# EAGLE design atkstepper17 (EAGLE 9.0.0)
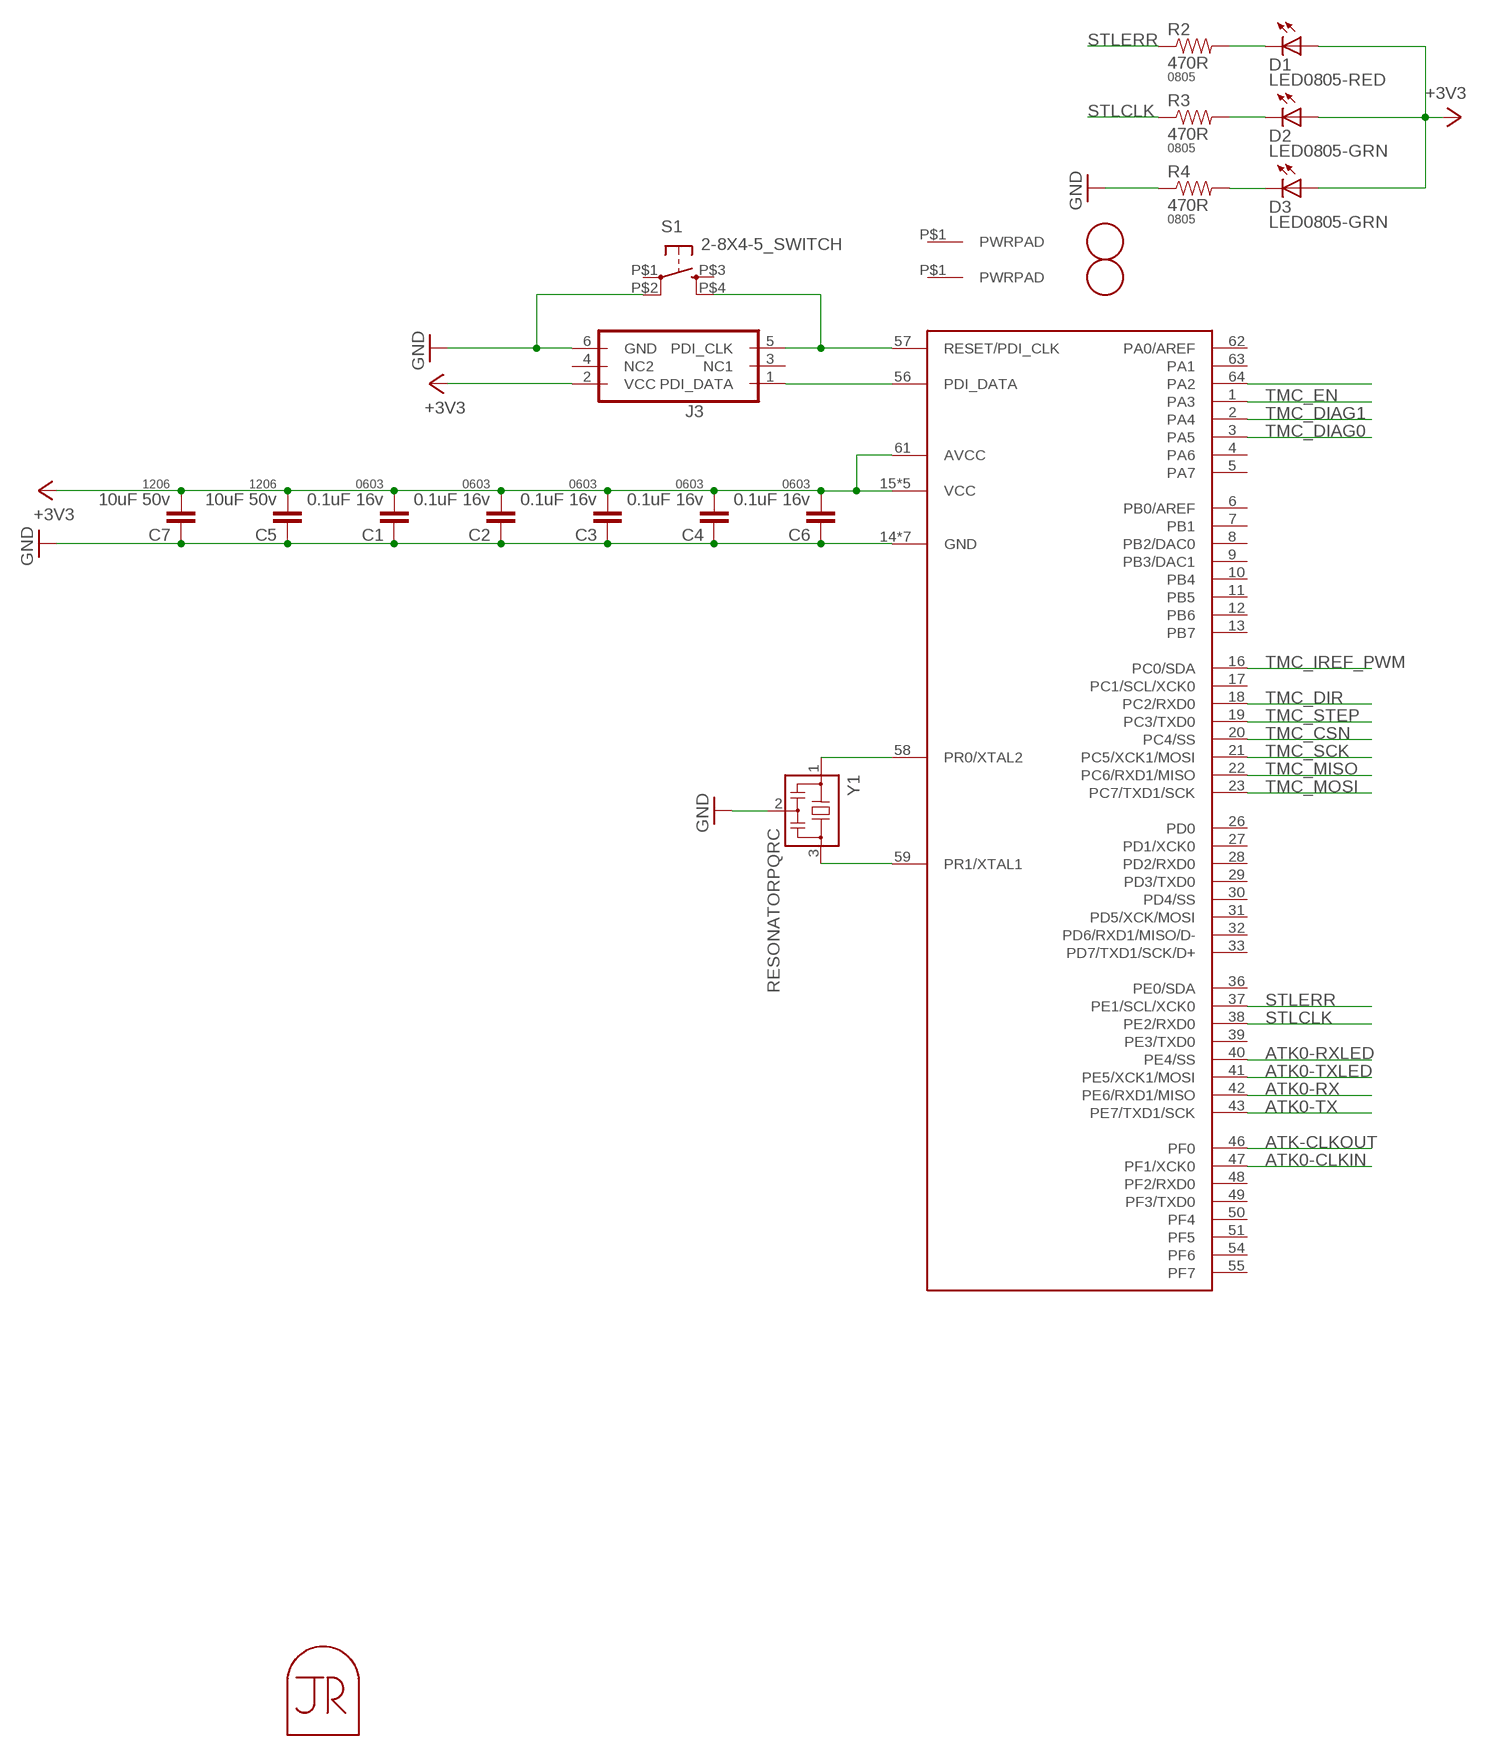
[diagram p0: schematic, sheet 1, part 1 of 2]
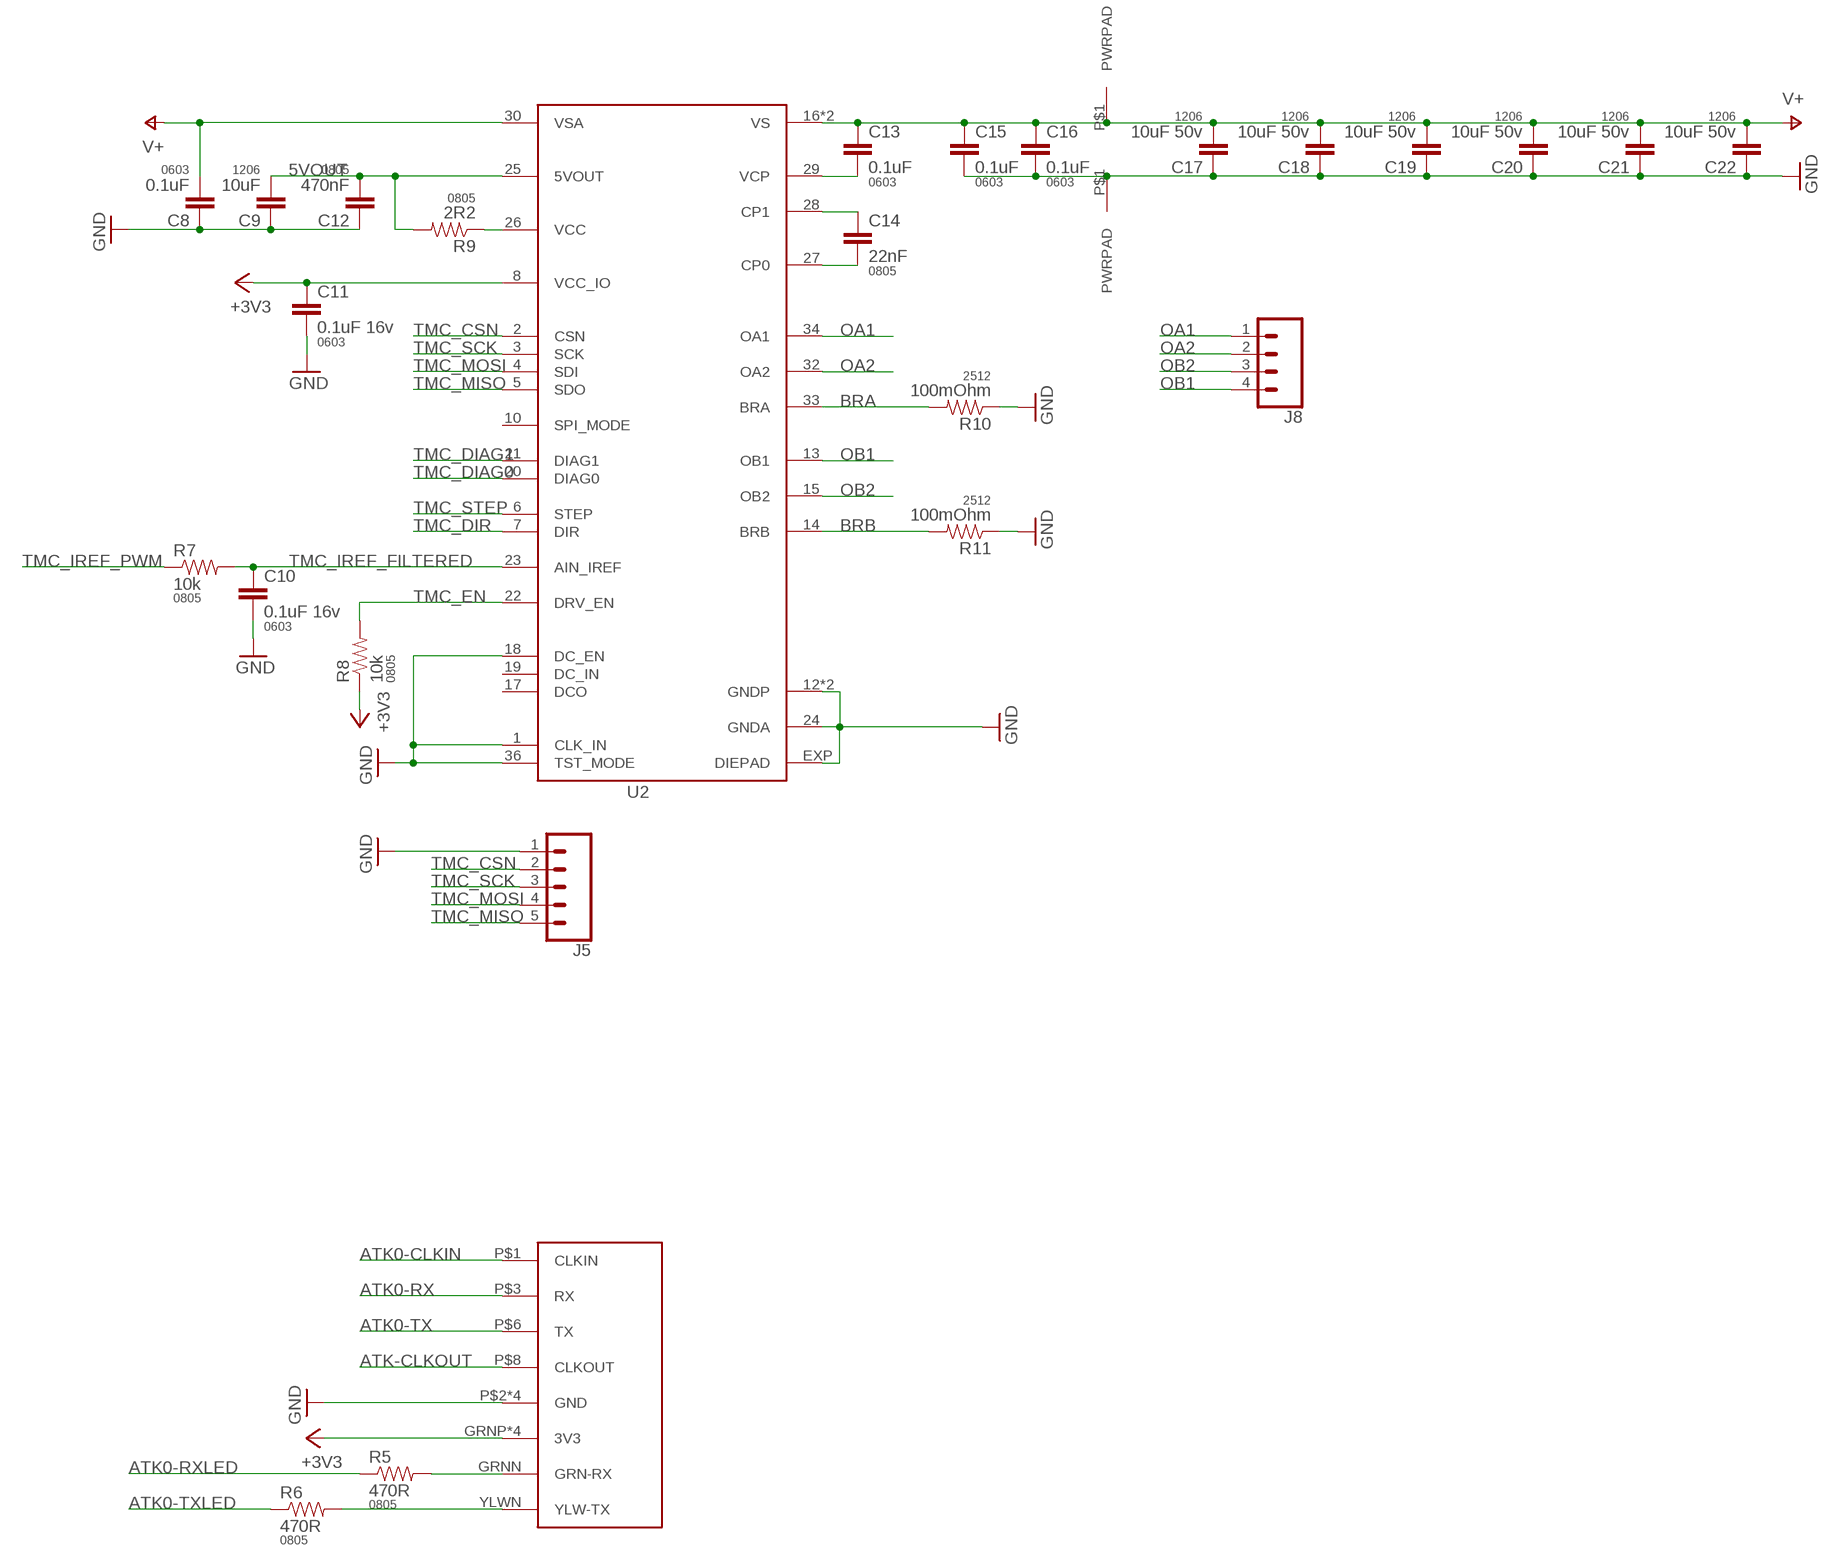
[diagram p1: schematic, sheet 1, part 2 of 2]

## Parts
C1  0.1uF 16v  CAP0603-CAP  [0603-CAP]
C2  0.1uF 16v  CAP0603-CAP  [0603-CAP]
C3  0.1uF 16v  CAP0603-CAP  [0603-CAP]
C4  0.1uF 16v  CAP0603-CAP  [0603-CAP]
C5  10uF 50v  CAP1206  [1206]
C6  0.1uF 16v  CAP0603-CAP  [0603-CAP]
C7  10uF 50v  CAP1206  [1206]
C8  0.1uF  CAP0603-CAP  [0603-CAP]
C9  10uF  CAP1206  [1206]
C10  0.1uF 16v  CAP0603-CAP  [0603-CAP]
C11  0.1uF 16v  CAP0603-CAP  [0603-CAP]
C12  470nF  CAP0805  [0805]
C13  0.1uF  CAP0603-CAP  [0603-CAP]
C14  22nF  CAP0805  [0805]
C15  0.1uF  CAP0603-CAP  [0603-CAP]
C16  0.1uF  CAP0603-CAP  [0603-CAP]
C17  10uF 50v  CAP1206  [1206]
C18  10uF 50v  CAP1206  [1206]
C19  10uF 50v  CAP1206  [1206]
C20  10uF 50v  CAP1206  [1206]
C21  10uF 50v  CAP1206  [1206]
C22  10uF 50v  CAP1206  [1206]
D1  LED0805-RED  LED0805  [LED0805]
D2  LED0805-GRN  LED0805  [LED0805]
D3  LED0805-GRN  LED0805  [LED0805]
J1  PWRPADM3  [PWRPAD_3-25MM]
J2  PWRPADM3  [PWRPAD_3-25MM]
J3  PDIFEMALE_SMD  [PDI_2X3_SMD]
J4  ATK-PHY  [RJ45-LED-RJE7318800XXX]
J5  CONN_05NO_SILK  [1X05_NO_SILK]
J6  PWRPAD  [PWRPAD_M3-PEM-MOUNT]
J7  PWRPAD  [PWRPAD_M3-PEM-MOUNT]
J8  CONN_04LONGPADS  [1X04_LONGPADS]
MP1  JRTOMBSTONE  [JRTOMBSTONE]
R2  470R  RESISTOR0805-RES  [0805]
R3  470R  RESISTOR0805-RES  [0805]
R4  470R  RESISTOR0805-RES  [0805]
R5  470R  RESISTOR0805-RES  [0805]
R6  470R  RESISTOR0805-RES  [0805]
R7  10k  RESISTOR0805-RES  [0805]
R8  10k  RESISTOR0805-RES  [0805]
R9  2R2  RESISTOR0805-RES  [0805]
R10  100mOhm  RESISTOR2512  [R2512]
R11  100mOhm  RESISTOR2512  [R2512]
S1  2-8X4-5_SWITCH  [TACT-SWITCH-KMR6]
U1  ATXMEGA_A3UQFN  [QFN-64-9X9MM]
U2  TMC2130  [QFN36-5X6]
U$1  FIDUCIAL  [FIDUCIAL_1MM]
U$2  FIDUCIAL  [FIDUCIAL_1MM]
Y1  RESONATORPQRC  [RES_PRQC]

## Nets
5VOUT: C9.2 C12.2 R9.2 U2.25(5VOUT)
+3V3: C1.2 C2.2 C3.2 C4.2 C5.2 C6.2 C7.2 C11.1 D1.1(A) D2.1(A) D3.1(A) J3.2(VCC) J4.GRNP(3V3) J4.P$4(3V3) J4.P$5(3V3) J4.YLWP(3V3) R8.1 U1.15(VCC) U1.25(VCC) U1.35(VCC) U1.45(VCC) U1.53(VCC) U1.61(AVCC) U2.8(VCC_IO)
ATK0-CLKIN: J4.P$1(CLKIN) U1.47(PF1/XCK0)
ATK0-RX: J4.P$3(RX) U1.42(PE6/RXD1/MISO)
ATK0-RXLED: R5.1 U1.40(PE4/SS)
ATK0-TX: J4.P$6(TX) U1.43(PE7/TXD1/SCK)
ATK0-TXLED: R6.1 U1.41(PE5/XCK1/MOSI)
ATK-CLKOUT: J4.P$8(CLKOUT) U1.46(PF0)
BRA: R10.2 U2.33(BRA)
BRB: R11.2 U2.14(BRB)
GND: C1.1 C2.1 C3.1 C4.1 C5.1 C6.1 C7.1 C8.1 C9.1 C10.2 C11.2 C12.1 C15.2 C16.2 C17.1 C18.1 C19.1 C20.1 C21.1 C22.1 J3.6(GND) J4.P$2(GND) J4.P$7(GND) J4.SHDL1(GND) J4.SHDL2(GND) J5.1 J7.P$1(PWRPAD) R4.1 R10.1 R11.1 S1.P$2(P1) U1.14(GND) U1.24(GND) U1.34(GND) U1.44(GND) U1.52(GND) U1.60(GND) U1.P$1(GND) U2.1(CLK_IN) U2.12(GNDP) U2.18(DC_EN) U2.24(GNDA) U2.35(GNDP) U2.36(TST_MODE) U2.EXP(DIEPAD) Y1.2
N$1: D3.2(C) R4.2
N$2: J3.5(PDI_CLK) S1.P$4(S1) U1.57(RESET/PDI_CLK)
N$3: U1.58(PR0/XTAL2) Y1.1
N$4: U1.59(PR1/XTAL1) Y1.3
N$5: D2.2(C) R3.2
N$6: D1.2(C) R2.2
N$8: J3.1(PDI_DATA) U1.56(PDI_DATA)
N$12: C14.2 U2.27(CP0)
N$13: R9.1 U2.26(VCC)
N$14: C14.1 U2.28(CP1)
N$15: C13.2 U2.29(VCP)
N$16: J4.GRNN(GRN-RX) R5.2
N$17: J4.YLWN(YLW-TX) R6.2
N$18: U1.64(PA2)
OA1: J8.1 U2.34(OA1)
OA2: J8.2 U2.32(OA2)
OB1: J8.4 U2.13(OB1)
OB2: J8.3 U2.15(OB2)
STLCLK: R3.1 U1.38(PE2/RXD0)
STLERR: R2.1 U1.37(PE1/SCL/XCK0)
TMC_CSN: J5.2 U1.20(PC4/SS) U2.2(CSN)
TMC_DIAG0: U1.3(PA5) U2.20(DIAG0)
TMC_DIAG1: U1.2(PA4) U2.21(DIAG1)
TMC_DIR: U1.18(PC2/RXD0) U2.7(DIR)
TMC_EN: R8.2 U1.1(PA3) U2.22(DRV_EN)
TMC_IREF_FILTERED: C10.1 R7.2 U2.23(AIN_IREF)
TMC_IREF_PWM: R7.1 U1.16(PC0/SDA)
TMC_MISO: J5.5 U1.22(PC6/RXD1/MISO) U2.5(SDO)
TMC_MOSI: J5.4 U1.23(PC7/TXD1/SCK) U2.4(SDI)
TMC_SCK: J5.3 U1.21(PC5/XCK1/MOSI) U2.3(SCK)
TMC_STEP: U1.19(PC3/TXD0) U2.6(STEP)
V+: C8.2 C13.1 C15.1 C16.1 C17.2 C18.2 C19.2 C20.2 C21.2 C22.2 J6.P$1(PWRPAD) U2.16(VS) U2.30(VSA) U2.31(VS)
Unconnected: J1.P$1(PWRPAD) J2.P$1(PWRPAD) J3.3(NC1) J3.4(NC2) S1.P$1(P) S1.P$3(S) U1.4(PA6) U1.5(PA7) U1.6(PB0/AREF) U1.7(PB1) U1.8(PB2/DAC0) U1.9(PB3/DAC1) U1.10(PB4) U1.11(PB5) U1.12(PB6) U1.13(PB7) U1.17(PC1/SCL/XCK0) U1.26(PD0) U1.27(PD1/XCK0) U1.28(PD2/RXD0) U1.29(PD3/TXD0) U1.30(PD4/SS) U1.31(PD5/XCK/MOSI) U1.32(PD6/RXD1/MISO/D-) U1.33(PD7/TXD1/SCK/D+) U1.36(PE0/SDA) U1.39(PE3/TXD0) U1.48(PF2/RXD0) U1.49(PF3/TXD0) U1.50(PF4) U1.51(PF5) U1.54(PF6) U1.55(PF7) U1.62(PA0/AREF) U1.63(PA1) U2.10(SPI_MODE) U2.17(DCO) U2.19(DC_IN)

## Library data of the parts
C1-C4 C6 C8 C10 C11 C13 C15 C16 = borkedlabs-passives:CAP: Capacitor; PACKAGE: 0603
C5 C7 C9 C17-C22 = borkedlabs-passives:CAP: Capacitor; PACKAGE: 1206
C12 C14 = borkedlabs-passives:CAP: Capacitor; PACKAGE: 0805
D1-D3 = lights:LED: LED
J1 J2 J6 J7 = power:PWRPAD
J3 = microcontrollers:PDI: Multi connection point. Often used as Generic Header-pin footprint for 0.1 inch spaced/style header connections You can populate with any combo of single row headers, but if you'd like an exact match, check these: Header - 2x3 (Male, 0.1") (PRT-12807) Header - 2x3 (Female, 0.1") (PRT-13010) 2x3 Pin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; PROD_ID: CONN-11290
J4 = connector:ATK-PHY
J5 = SparkFun-Connectors:CONN_05: Multi connection point. Often used as Generic Header-pin footprint for 0.1 inch spaced/style header connections On any of the 0.1 inch spaced packages, you can populate with these: Break Away Headers - Straight (PRT-00116) Break Away Male Headers - Right Angle (PRT-00553) Female Headers (PRT-00115)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
J8 = SparkFun-Connectors:CONN_04: Multi connection point. Often used as Generic Header-pin footprint for 0.1 inch spaced/style header connections On any of the 0.1 inch spaced packages, you can populate with these: Break Away Headers - Straight (PRT-00116) Break Away Male Headers - Right Angle (PRT-00553) Female Headers (PRT-00115)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; PROD_ID: CONN-09696
MP1 = connector:JRTOMBSTONE
R2-R9 = borkedlabs-passives:RESISTOR: Resistor; PACKAGE: 0805
R10 R11 = borkedlabs-passives:RESISTOR: Resistor; PACKAGE: 2512
S1 = fab:2-8X4-5_SWITCH
U1 = microcontrollers:ATXMEGA_A3U
U2 = power:TMC2130
U$1 U$2 = connector:FIDUCIAL: For use by pick and place machines to calibrate the vision/machine, 1mm
Y1 = passives:RESONATOR

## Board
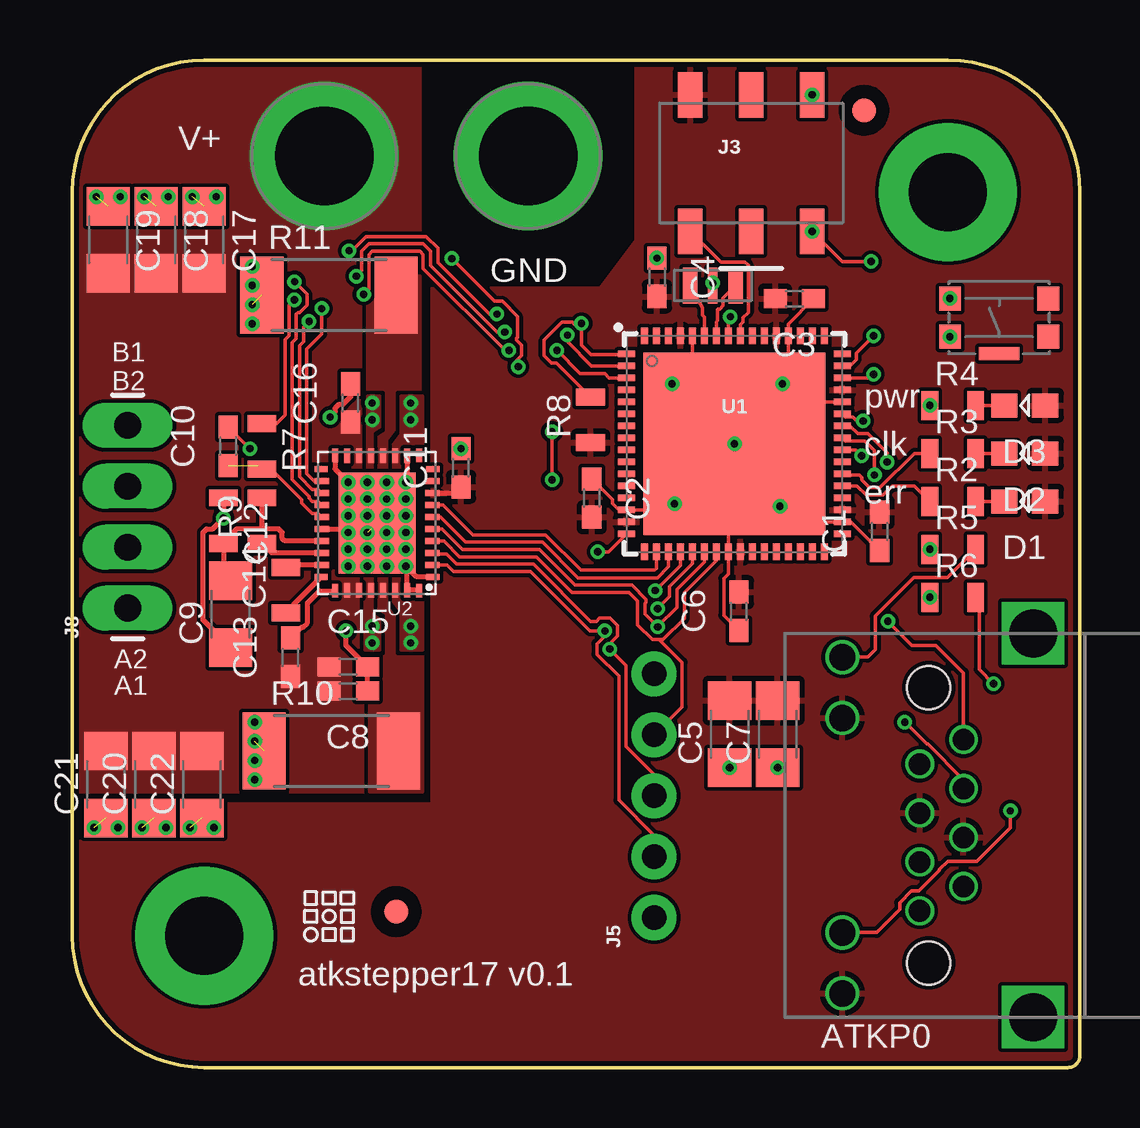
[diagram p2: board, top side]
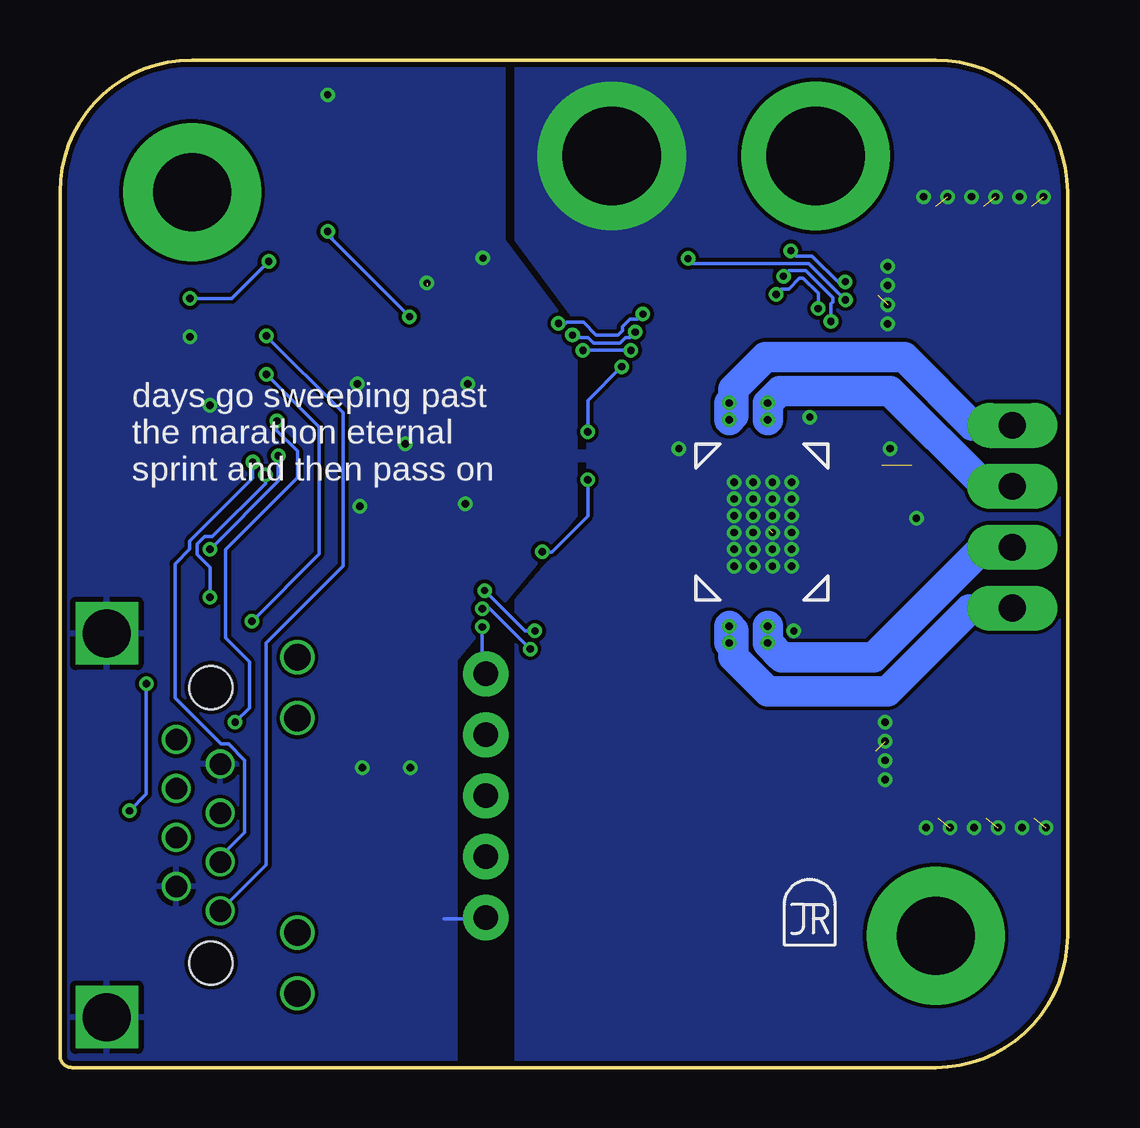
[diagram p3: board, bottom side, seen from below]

Size 42 x 42 mm. Coordinates in mm from the lower left corner, seen from the top.
Outline: 36.5,42 5.5,42 arc90 0,36.5 0,5.5 arc90 5.5,0 41.5,0 arc90 42,0.5 42,36.5 arc90 36.5,42
Copper layers (1*16): Top 0.035mm / dielectric 1.5mm / Bottom 0.035mm
Design rules "default *": minimum track width 6mil, minimum drill 0.3mm, track to track 6mil, track to pad 6mil, pad to pad 6mil, via to via 6mil, smd to smd 6mil, copper to edge 8mil, drill to drill 8mil, minimum pad ring 6mil, minimum via ring 6mil, stop-mask expansion 4mil, vias tented up to drill 27mil, thermal gap 9mil

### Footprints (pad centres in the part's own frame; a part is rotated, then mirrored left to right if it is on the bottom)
0603-CAP = smd 0.96 x 0.8: 1 -0.8,0; 2 0.8,0
1206 = smd 1.6 x 1.8: 1 -1.4,0; 2 1.4,0
0805 = smd 0.7 x 1.2: 1 -0.95,0; 2 0.95,0
LED0805 = smd 1.1 x 1: 1 -0.85,0; 2 0.85,0
PWRPAD_3-25MM = drill 3.25 pad 5.75: P$1 0,0
PDI_2X3_SMD = smd 1.02 x 1.9: 1 -2.54,-2.85; 2 -2.54,2.85; 3 0,-2.85; 4 0,2.85; 5 2.54,-2.85; 6 2.54,2.85
RJ45-LED-RJE7318800XXX = drill 1.1: GRNN 7.01,3.6; GRNP 4.47,3.6; YLWN -4.47,3.6; YLWP -7.01,3.6 | drill 0.9: P$1 -3.57,0.38; P$2 -2.55,-1.45; P$3 -1.53,0.38; P$4 -0.51,-1.45; P$5 0.51,0.38; P$6 1.53,-1.45; P$7 2.55,0.38; P$8 3.57,-1.45 | drill 2 square: SHDL1 -8,-4.35; SHDL2 8,-4.35 | hole 1.8: -5.74,0; 5.74,0
1X05_NO_SILK = drill 1.016 pad 1.88: 1 0,0; 2 2.54,0; 3 5.08,0; 4 7.62,0; 5 10.16,0
PWRPAD_M3-PEM-MOUNT = drill 4.1 pad 6.2: P$1 0,0
1X04_LONGPADS = drill 1.118 pad 1.88 long: 1 0,0; 2 2.54,0; 3 5.08,0; 4 7.62,0
R2512 = smd 1.8 x 3.2: 1 -2.8,0; 2 2.8,0
TACT-SWITCH-KMR6 = smd 0.9 x 1: P$1 -2.05,0.8; P$2 2.05,0.8; P$3 -2.05,-0.8; P$4 2.05,-0.8 | smd 1.7 x 0.55: P$5 0,1.5
QFN-64-9X9MM = smd 0.7 x 0.275: 1 -4.5,3.75; 2 -4.5,3.25; 3 -4.5,2.75; 4 -4.5,2.25; 5 -4.5,1.75; 6 -4.5,1.25; 7 -4.5,0.75; 8 -4.5,0.25; 9 -4.5,-0.25; 10 -4.5,-0.75; 11 -4.5,-1.25; 12 -4.5,-1.75; 13 -4.5,-2.25; 14 -4.5,-2.75; 15 -4.5,-3.25; 16 -4.5,-3.75; 33 4.5,-3.75; 34 4.5,-3.25; 35 4.5,-2.75; 36 4.5,-2.25; 37 4.5,-1.75; 38 4.5,-1.25; 39 4.5,-0.75; 40 4.5,-0.25; 41 4.5,0.25; 42 4.5,0.75; 43 4.5,1.25; 44 4.5,1.75; 45 4.5,2.25; 46 4.5,2.75; 47 4.5,3.25; 48 4.5,3.75 | smd 0.275 x 0.7: 17 -3.75,-4.5; 18 -3.25,-4.5; 19 -2.75,-4.5; 20 -2.25,-4.5; 21 -1.75,-4.5; 22 -1.25,-4.5; 23 -0.75,-4.5; 24 -0.25,-4.5; 25 0.25,-4.5; 26 0.75,-4.5; 27 1.25,-4.5; 28 1.75,-4.5; 29 2.25,-4.5; 30 2.75,-4.5; 31 3.25,-4.5; 32 3.75,-4.5; 49 3.75,4.5; 50 3.25,4.5; 51 2.75,4.5; 52 2.25,4.5; 53 1.75,4.5; 54 1.25,4.5; 55 0.75,4.5; 56 0.25,4.5; 57 -0.25,4.5; 58 -0.75,4.5; 59 -1.25,4.5; 60 -1.75,4.5; 61 -2.25,4.5; 62 -2.75,4.5; 63 -3.25,4.5; 64 -3.75,4.5 | smd 7.6 x 7.6: P$1 0,0
QFN36-5X6 = smd 0.55 x 0.25: 1 -2.325,1.75; 10 -2.325,-2.75; 19 2.325,-2.75; 28 2.325,1.75 | smd 0.6 x 0.25: 2 -2.3,1.25; 3 -2.3,0.75; 4 -2.3,0.25; 5 -2.3,-0.25; 6 -2.3,-0.75; 7 -2.3,-1.25; 8 -2.3,-1.75; 9 -2.3,-2.25; 20 2.3,-2.25; 21 2.3,-1.75; 22 2.3,-1.25; 23 2.3,-0.75; 24 2.3,-0.25; 25 2.3,0.25; 26 2.3,0.75; 27 2.3,1.25 | smd 0.25 x 0.55: 11 -1.75,-3.325; 18 1.75,-3.325; 29 1.75,2.325; 36 -1.75,2.325 | smd 0.25 x 0.6: 12 -1.25,-3.3; 13 -0.75,-3.3; 14 -0.25,-3.3; 15 0.25,-3.3; 16 0.75,-3.3; 17 1.25,-3.3; 30 1.25,2.3; 31 0.75,2.3; 32 0.25,2.3; 33 -0.25,2.3; 34 -0.75,2.3; 35 -1.25,2.3 | smd 3.2 x 4.2: EXP 0,-0.5
FIDUCIAL_1MM = smd 1 x 1: 1 0,0
RES_PRQC = smd 0.6 x 1.5: 1 -0.95,0; 3 0.95,0 | smd 0.4 x 1.5: 2 0,0

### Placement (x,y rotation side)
C1  33.65,22.35 90 top
C2  21.65,23.74 270 top
C3  30.1,32.05 180 top
C4  24.37,32.95 270 top
C5  27.4,13.9 90 top
C6  27.79,19.02 90 top
C7  29.4,13.9 90 top
C8  11.5,15.7 180 top
C9  6.6,18.9 90 top
C10  6.5,25.9 90 top
C11  16.2,25 90 top
C12  6.3,22.8 270 top
C13  9.1,17.1 90 top
C14  8.9,19.9 90 top
C15  11.5,16.7 0 top
C16  11.6,27.7 90 top
C17  5.5,34.5 270 top
C18  3.5,34.5 270 top
C19  1.5,34.5 270 top
C20  3.4,11.8 90 top
C21  1.4,11.8 90 top
C22  5.4,11.8 90 top
D1  39.7,23.6 180 top
D2  39.7,25.6 180 top
D3  39.7,27.6 180 top
J1  5.5,5.5 180 top
J2  36.5,36.5 180 top
J3  28.3,37.7 0 top
J4  35.7,10.1 90 top
J5  24.25,6.25 90 top
J6  10.5,38 180 top
J7  19,38 180 top
J8  2.3,19.15 90 top
MP1  10.7,6.1 0 bottom
R2  36.7,23.6 0 top
R3  36.7,25.6 0 top
R4  36.7,27.6 0 top
R5  36.7,21.6 0 top
R6  36.7,19.6 0 top
R7  7.9,25.9 270 top
R8  21.6,27 90 top
R9  7.9,22.8 90 top
R10  10.8,13.2 0 top
R11  10.7,32.2 0 top
S1  38.63,31.26 180 top
U1  27.6,26 0 top
U2  12.7,22.2 180 top
U$1  13.5,6.5 0 top
U$2  33,39.9 0 top
U$5  [CBA-SILK-LOGO]  10.7,6.3 90 top
Y1  26.7,32.6 180 top

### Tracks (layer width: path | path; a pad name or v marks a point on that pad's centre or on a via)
5VOUT
  Top 0.203: C12.2 6.2,21.65 | C12.2 6.3,21.9 6.85,22.45 7.9,22.45 | C12.2 6.3,20.6 C9.2 | U2.25 8.85,21.95 8.75,22.05 8.75,22.3 8.61,22.45 7.9,22.45 | R9.2 7.9,22.45
+3V3
  Top 0.203: U2.8 15.95,23.95 C11.1
  pour Top: -3,11 15,11 15,32.5 22,32.5 23.5,34.5 23.5,43 43,43 43,-2 -3,-2
ATK0-CLKIN  (via drill 0.3)
  Top 0.152: v33.4,30.5 32.68,29.78 32.68,29.52 32.41,29.25 U1.47
  Bottom 0.152: v33.4,30.5 30.2,27.3 30.2,20.9 33.4,17.7 33.4,8.45 J4.P$1
ATK0-RX  (via drill 0.3)
  Top 0.152: U1.42 32.41,26.75 32.74,26.42 33.17,26.42 33.97,25.62 v33.97,25.24
  Bottom 0.152: v33.97,25.24 33.97,24.57 36.59,21.95 36.59,21.61 37.2,21 37.2,15.4 35.28,13.48 34.98,13.48 34.3,12.8 34.3,9.8 35.32,8.78 J4.P$3
ATK0-RXLED  (via drill 0.3)
  Top 0.152: U1.40 32.66,25.75 v32.91,25.5
  Bottom 0.152: v32.91,25.5 32.91,24.45 R5.1
  other vias: 35.75,21.6
ATK0-TX  (via drill 0.3)
  Top 0.152: U1.43 32.23,27.12 32.55,27.12 32.71,26.95 v32.96,26.95 | v34.7,14.4 35.62,13.48 35.66,13.48 37.15,11.99 J4.P$6
  Bottom 0.152: v32.96,26.95 32.96,26.56 32.1,25.7 32.1,24.6 35.1,21.6 35.1,17.9 34.1,16.9 34.1,15 v34.7,14.4
ATK0-TXLED  (via drill 0.3)
  Top 0.152: U1.41 32.23,26.12 33.04,26.12 33.44,25.72 v33.44,24.7
  Bottom 0.152: v33.44,24.7 33.44,24.34 35.65,22.13 35.97,22.13 36.28,21.82 36.28,21.38 35.75,20.85 R6.1
  other vias: 35.75,19.6
ATK-CLKOUT  (via drill 0.3)
  Top 0.152: U1.46 33.25,28.75 v33.4,28.9 | v34,18.6 35,17.6 36,17.6 37.15,16.45 J4.P$8
  Bottom 0.152: v33.4,28.9 31.2,26.7 31.2,21.4 v34,18.6
BRA
  pour Top (rank 4, no thermals): 14.6,20.6 14.6,11.5 12.4,11.5 12.4,20.6
BRB
  pour Top (rank 4, no thermals): 14.5,33 14.5,23.9 12.3,23.9 12.3,33
GND  (via drill 0.3)  (10 unrouted)
  Top 0.152: 13.95,20.95 v13.9,20.9 | 13.95,23.95 U2.EXP | R4.1 35.85,27.7 | C10.2 v7.4,25.8 | U1.60 25.85,29.35 25.8,29.3 25.8,27.8 27.55,26.05 | 27.55,26.05 U1.P$1 27.45,25.85 | 29.45,27.95 29.85,28.35 U1.52 29.85,31 C3.1 | 29.45,27.95 27.55,26.05 | 27.35,25.75 v25.1,23.5 24.85,23.25 U1.14 22.79,23.25 22.52,23.52 22.52,23.67 C2.1 | 27.35,25.75 U1.24 27.35,20.58 27.16,20.39 27.16,18.85 C6.1 | 27.35,25.75 27.45,25.85 | 27.45,25.85 30.55,22.75 U1.34 32.45,22.75 C1.1 | U1.44 29.65,27.75 29.45,27.95
  Top 0.203: U2.24 12.45,22.45 U2.EXP | C9.1 5.45,18.65 5.45,22.3 5.59,22.45 5.85,22.45 v6.3,22.9 C12.1 | U2.12 13.95,24.45 v13.9,24.4 | 13.95,20.85 U2.35 14.43,19.9 U2.36 | 13.95,20.85 v13.9,20.9 | U2.1 14.35,20.45 13.95,20.85 | U2.18 10.95,24.95 v11.5,24.4 | C16.2 11.6,27.96 11.27,27.63 11.1,27.63 10.95,27.48 10.95,27.31 v10.74,27.11 | C8.1 C15.2 11.41,17.59 v11.41,18.2
  Bottom 0.152: J5.1 24.3,6.2 26,6.2
  other vias: 11.5,21.6 12.3,21.6 13.1,21.6 13.9,21.6 13.1,23.7 13.1,23 13.9,23.7 13.9,23 12.3,23 12.3,23.7 11.5,23.7 11.5,23 13.9,22.3 13.1,22.3 12.3,22.3 11.5,22.3 13.1,24.4 12.3,24.4 11.5,20.9 12.3,20.9 13.1,20.9 7.6,12 7.6,12.8 7.6,14.4 7.6,13.6 5.9,10 4.9,10 3.9,10 2.9,10 1.9,10 0.9,10 6,36.3 5,36.3 4,36.3 3,36.3 2,36.3 1,36.3 7.5,33.4 7.5,31 7.5,32.6 7.5,31.8 35.75,27.6 36.58,30.46 24.37,33.75 26.7,32.7 27.6,26 29.5,23.4 25,28.5 29.6,28.5 30.84,40.55 29.4,12.5 27.4,12.5 16.2,25.8
  pour Bottom: -2.5,-1.5 23,-1.5 23,19.5 20,23 20,25.3 20.5,25.3 20.5,25.7 20,25.7 20.1,30.6 23,34.5 23,44.5 -2.5,44.5
  pour Bottom: 25.5,-2.5 25.5,17 20.5,23 20.5,30.5 23.5,34.5 23.5,43 43.5,43 43.5,-2.5
N$1
  Top 0.152: D3.2 R4.2
N$2  (via drill 0.3)
  Top 0.152: 27.4,30.55 U1.57 27.35,31.22 v27.43,31.3 | J3.5 32.09,33.6 v33.3,33.6
  Bottom 0.152: 30.65,34.55 30.81,34.8 | 30.81,34.8 J3.5 | v27.43,31.3 30.81,34.67 30.81,34.8 | v33.3,33.6 34.84,32.06 S1.P$4
  other vias: 30.84,34.85 36.58,32.06
N$3
  Top 0.152: U1.58 26.85,31.08 26.9,31.13 26.9,31.6 26.92,31.62 27,31.62 27.13,31.75 27.13,32.08 Y1.1
N$4
  Top 0.152: Y1.3 26.27,31.68 26.27,31.36 26.35,31.28 U1.59
N$5
  Top 0.152: D2.2 R3.2
N$6
  Top 0.152: D1.2 R2.2
N$8
  Top 0.152: J3.1 27.03,33.58 28.05,33.58 28.18,33.45 28.18,31.48 27.96,31.26 27.96,31.08 27.85,30.97 U1.56
N$12
  Top 0.203: U2.27 9.3,20.95 C14.2
N$13
  Top 0.203: R9.1 8.3,21.45 8.49,21.45 9.9,21.45 9.91,21.45 U2.26
N$14
  Top 0.203: U2.28 9.2,19.27 C14.1
N$15
  Top 0.203: C13.2 9.55,18.35 9.61,18.35 9.8,18.54 9.8,19.37 10.3,19.88 U2.29
N$16
  Top 0.152: J4.GRNN 33.16,17.11 33.47,17.42 33.47,18.82 35.08,20.43 36.48,20.43 R5.2
N$17  (via drill 0.3)
  Top 0.152: R6.2 37.8,19.45 37.8,16.6 v38.4,16 | v39.1,10.7 39.1,10 37.7,8.6 36.5,8.6 36.15,8.25 36.15,8.23 35.29,7.36 34.98,7.36 34.49,6.87 34.49,6.59 33.53,5.63 J4.YLWN
  Bottom 0.152: v38.4,16 38.4,11.4 v39.1,10.7
OA1  (via drill 0.3)
  Bottom 1.27: 13.92,17.52 v14.1,17.7 v14.1,18.4 13.92,18.22 13.92,17.11 12.49,15.68 7.51,15.68 4.09,19.1 2.35,19.1 J8.1
  pour Top (no thermals): 13.7,20.6 13.7,19.4 14.6,19.4 14.6,17.4 13.7,17.4 13.7,19 13.4,19.4 13.4,20.6
OA2  (via drill 0.3)
  Bottom 1.27: J8.2 2.51,21.7 3.5,21.7 8.1,17.1 11.9,17.1 v12.5,17.7 v12.5,18.4
  pour Top (no thermals): 12.5,20.6 12.5,18.9 12.8,18.7 12.8,17.4 12.2,17.4 12.2,20.6
OB1  (via drill 0.3)
  Bottom 1.27: v14.1,27.7 v14.1,27 13.92,27.18 13.92,28.29 12.59,29.62 6.81,29.62 3.96,26.77 J8.4
  pour Top (no thermals): 13.7,24.8 13.7,26 14.6,26 14.6,28 13.7,28 13.7,26.4 13.4,26 13.4,24.8
OB2  (via drill 0.3)
  Bottom 1.27: v12.5,27 v12.5,27.7 12,28.2 9.1,28.2 7.4,28.2 3.43,24.23 J8.3
  pour Top (no thermals): 12.5,24.8 12.5,26.5 12.8,26.7 12.8,28 12.3,28 12.3,24.8
STLCLK
  Top 0.152: U1.38 32.15,24.7 32.8,24.7 32.91,24.59 32.91,24.48 33.22,24.17 33.67,24.17 35.1,25.6 R3.1
STLERR
  Top 0.152: R2.1 35.1,24.25 34.18,24.25 33.8,23.86 33.09,23.86 32.7,24.25 U1.37
TMC_CSN  (via drill 0.3)
  Top 0.152: U2.2 15.63,20.95 15.89,20.68 19.09,20.68 21.58,18.2 v22.2,18.2 22.2,17.99 21.87,17.66 21.87,17.22 22.78,16.32 22.78,11.15 24.25,9.68 J5.2 | U1.20 25.35,20.93 v24.3,19.89
  Bottom 0.152: v24.3,19.89 22.61,18.2 v22.2,18.2
TMC_DIAG0  (via drill 0.3)
  Top 0.152: U2.20 10.08,24.45 9.78,24.75 9.78,29.96 10.39,30.58 v10.39,31.64 | v18.2,29.9 18.03,29.9 14.63,33.3 14.63,33.9 14.49,34.03 12.51,34.03 12.37,33.9 12.37,32.46 v12.14,32.23 | v20.2,29.9 21.17,28.93 22.2,28.93 22.37,28.75 U1.3
  Bottom 0.152: v18.2,29.9 v20.2,29.9 | v10.39,31.64 10.39,32.28 11.03,32.91 11.17,32.91 11.62,32.46 11.92,32.46 v12.14,32.23
TMC_DIAG1  (via drill 0.3)
  Top 0.152: U2.21 10.25,24.1 10,24.1 9.47,24.63 9.47,30.08 9.64,30.25 9.64,30.87 v9.86,31.1 | v18.02,30.66 17.7,30.66 14.93,33.43 14.93,34.02 14.62,34.33 12.38,34.33 12.07,34.02 12.07,33.21 v11.84,32.99 | U1.2 21.65,29.25 20.64,30.27 v20.64,30.54
  Bottom 0.152: v18.02,30.66 18.25,30.43 18.42,30.43 18.65,30.2 19.75,30.2 19.98,30.43 20.53,30.43 v20.64,30.54 | v9.86,31.1 9.86,31.84 9.79,31.91 9.79,32.1 10.9,33.21 11.61,33.21 v11.84,32.99
TMC_DIR
  Top 0.152: U2.7 15.45,23.45 16.7,22.2 19.73,22.2 21.2,20.73 24.27,20.73 24.35,20.81 U1.18
TMC_EN  (via drill 0.3)
  Top 0.152: U2.22 10.25,23.6 10.01,23.6 9.87,23.73 9.87,23.8 9.16,24.5 9.16,30.21 9.33,30.38 9.33,31.4 9.4,31.47 9.47,31.47 9.79,31.78 9.79,32.23 v9.26,32.76 | v17.7,31.41 17.38,31.41 15.24,33.55 15.24,34.15 14.75,34.64 12.25,34.64 11.66,34.05 v11.54,34.05 | v21.22,31.02 21.22,31 | 21.22,31 21.22,30.11 21.62,29.72 23.07,29.72 U1.1 | 21.22,31 20.92,31 20.86,31.07 20.41,31.07 19.67,30.32 19.67,29.68 19.98,29.37 20.18,29.37 R8.2
  Bottom 0.152: v17.7,31.41 17.92,31.19 18.24,31.19 18.55,30.88 18.55,30.73 18.74,30.54 19.66,30.54 20.18,31.07 20.86,31.07 20.9,31.02 v21.22,31.02 | v9.26,32.76 9.58,32.76 10.61,33.79 10.65,33.82 11.32,33.82 11.54,34.04 v11.54,34.05
TMC_IREF_FILTERED  (1 unrouted)
  Top 0.152: U2.23 10.25,23.1 10.01,23.1 9.57,23.54 9.57,23.67 8.29,24.95 R7.2 7.75,25.1
TMC_IREF_PWM  (via drill 0.3)
  Top 0.152: R7.1 8.51,26.85 8.86,27.2 8.86,30.34 9.03,30.5 9.03,31.77 v9.26,32 | v15.82,33.72 17.6,31.94 17.92,31.94 18.55,31.31 18.55,30.44 18.52,30.41 18.52,30.32 18.73,30.12 18.73,29.68 18.52,29.48 18.52,29.27 v18.59,29.21 | v21.9,21.5 22.35,21.5 U1.16 | v20,26.5 v20,24.5
  Bottom 0.152: v18.59,29.21 20,27.8 v20,26.5 | v21.9,21.5 21.5,21.5 20,23 v20,24.5 | v15.82,33.72 15.62,33.52 10.77,33.52 v9.26,32
TMC_MISO  (via drill 0.3)
  Top 0.152: U2.5 15.42,22.45 16.27,21.59 19.47,21.59 20.96,20.11 23.32,20.11 23.92,19.52 23.92,19.39 23.87,19.35 23.87,18.91 v24.4,18.38 | v24.4,18.38 v24.4,18.37 | v24.4,18.38 25.2,19.18 25.2,19.93 26.35,21.07 U1.22
  Bottom 0.152: v24.4,18.37 24.4,16.56 J5.5
TMC_MOSI
  Top 0.152: U2.4 15.49,21.95 16.15,21.29 19.35,21.29 20.83,19.81 23.2,19.81 23.56,19.44 23.56,18.45 24.18,17.84 24.5,17.84 | 24.5,17.84 24.62,17.84 25.51,18.73 25.51,19.8 26.85,21.14 U1.23 | 24.5,17.84 24.5,17.81 25.42,16.89 25.42,15.04 J5.4
TMC_SCK  (via drill 0.3)
  Top 0.152: U2.3 15.05,21.4 15.61,21.4 16.02,20.99 19.22,20.99 21.6,18.6 21.85,18.6 21.98,18.73 22.42,18.73 22.73,18.42 22.73,17.98 22.4,17.65 v22.4,17.44 23.08,16.76 23.08,13.39 24.25,12.22 J5.3 | U1.21 25.85,21 24.9,20.05 24.9,19.63 v24.4,19.13
  Bottom 0.152: v22.4,17.44 24.09,19.13 v24.4,19.13
TMC_STEP
  Top 0.152: U2.6 15.35,22.95 16.4,21.9 19.6,21.9 21.08,20.42 24.38,20.42 24.85,20.88 U1.19
V+
  pour Top (rank 5, no thermals): -2.5,11.5 14.5,11.5 14.4,32.6 14.5,33 14.5,42.6 13.9,43 -2.5,43

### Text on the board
tPlace: V+ | GND | B1 | B2 | pwr | clk | err | A2 | A1 | atkstepper17 v0.1 | ATKP0
bPlace: days go sweeping past / the marathon eternal / sprint and then pass on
